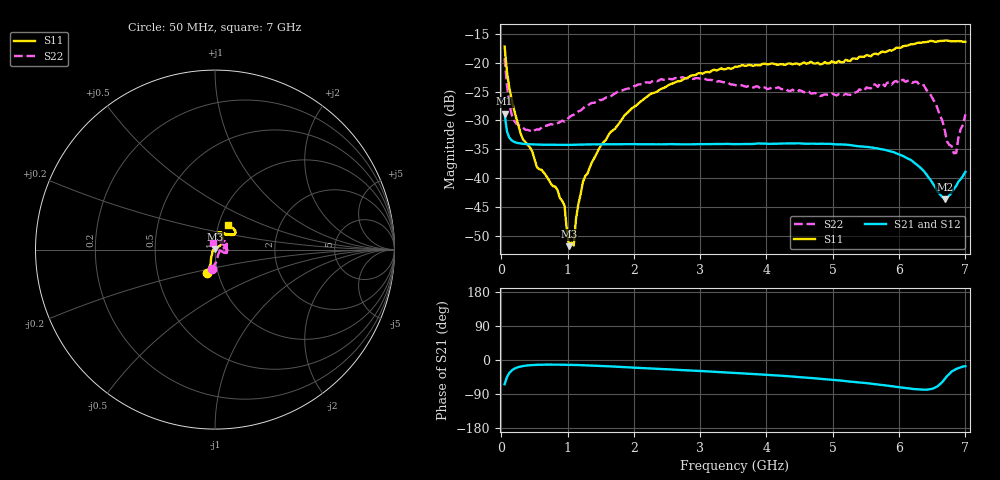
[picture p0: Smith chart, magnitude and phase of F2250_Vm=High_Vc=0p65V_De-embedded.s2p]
! Integrated Device Technology
! Corporate Headquarters
! 6024 Silver Creek Valley Road
! San Jose, CA 95138  USA
! Phone:  1-408-284-8200
! Toll Free:  1-800-223-1366
! Webpage:  http://www.idt.com/
! Timing and RF Division
! 515 Groton Road, Suite 102
! Westford, MA 01886-6024
! Device:  F2250
! Description: Voltage Variable RF Attenuator
! Frequency:  50.0 -  6000.00 MHz
! Package:  3x3 mm Thin QFN Plastic Package: 16 pin
! Ports:  2 RF, 3 DC
!  Pin  1  = GND
!  Pin  2  = NC
!  Pin  3  = RF1  = Port 1
!  Pin  4  = NC
!  Pin  5  = GND
!  Pin  6  = GND
!  Pin  7  = GND
!  Pin  8  = GND
!  Pin  9  = NC
!  Pin 10  = RF2  = Port 2
!  Pin 11  = NC
!  Pin 12  = GND
!  Pin 13  = GND
!  Pin 14  = VCNTRL
!  Pin 15  = VDD
!  Pin 16  = VMODE
! Vcntrl:  0.650 Volts
! Vmode:  +3.300 Volts
! Vdd:  +3.30  Volts
! Current:  1.282 mA
! Data:  The device was measured on a the F2250 evaluation board which has
!  individual transmission lines to the RF pins.  Data was collected
!  using a calibrated network analyzer.  The evaluation board was
!  de-embedded using a TRL calibration technique.
!  The reference plane is the edge of the package pin.
! Misc:  SN 10
!  Action Tracker AT0258
! Date Measured:  2014-11-26
! Date:  2015-10-15  MJV
! Note:
!  Integrated Device Technology supplies this data as a sample of measured
!  data at the package pin for this product.  Your particular data for this
!  product may vary.
!  Data was taken at 25 degrees C.
!  Integrated Device Technology reserves the right to change this data at anytime.
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# GHz S dB R 50
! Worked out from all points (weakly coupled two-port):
!   201 points, 50 MHz to 7 GHz, reference 50 ohm
!   highest |S21| = -28.81 dB at 50 MHz (marker M1); lowest = -43.7 dB at 6.687 GHz (marker M2)
!   lowest |S11| = -51.8 dB at 1.023 GHz (marker M3), VSWR 1.01, Z = 49.8 + j0.172 ohm
!   |S11| at or under -10 dB: start of sweep to end of sweep
!   |S22| runs from -35.7 to -19.2 dB; largest |S21 - S12| = 6.3e-05
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0.05  -17.17 -108.3  -28.81 -64.0  -28.81 -64.0  -19.20 -99.3
0.1195  -24.20 -111.6  -32.95 -34.6  -32.94 -34.6  -26.90 -70.8
0.22375  -29.45 -121.8  -33.84 -20.8  -33.83 -20.8  -30.51 -47.2
0.5365  -38.09 -153.6  -34.17 -12.7  -34.17 -12.7  -31.55 -9.8
0.8145  -41.46 170.6  -34.22 -12.2  -34.22 -12.2  -30.65 -1.3
0.9535  -44.77 171.5  -34.23 -12.5  -34.23 -12.5  -30.21 0.4
1.023  -51.81 137.7  -34.23 -12.7  -34.23 -12.7  -29.45 2.1
1.0925  -51.70 83.0  -34.22 -13.0  -34.21 -13.0  -29.01 3.5
1.12725  -47.04 56.6  -34.21 -13.2  -34.21 -13.2  -28.68 2.8
1.2315  -40.66 38.5  -34.17 -13.7  -34.17 -13.7  -27.89 2.2
1.6485  -31.98 40.4  -34.12 -16.9  -34.13 -16.9  -25.82 10.3
2.37825  -24.75 46.3  -34.13 -23.4  -34.13 -23.4  -23.05 20.7
3.525  -20.67 71.5  -34.10 -34.1  -34.10 -34.1  -23.83 48.6
4.7065  -20.09 71.9  -34.02 -48.0  -34.02 -48.0  -25.27 53.9
5.2625  -19.68 53.1  -34.26 -57.0  -34.26 -57.1  -25.56 29.1
5.85325  -17.81 40.4  -35.31 -68.4  -35.31 -68.4  -23.36 0.8
6.3745  -16.41 40.8  -38.79 -78.4  -38.79 -78.4  -23.89 -15.8
6.54825  -16.36 44.6  -41.66 -72.4  -41.67 -72.6  -27.01 -18.1
6.68725  -16.13 47.7  -43.69 -50.4  -43.69 -50.3  -31.58 0.5
6.722  -16.11 49.2  -43.43 -42.6  -43.41 -42.5  -33.62 6.1
6.861  -16.23 54.4  -41.35 -23.8  -41.33 -23.7  -35.63 64.3
7  -16.35 62.3  -38.92 -16.4  -38.89 -16.6  -28.93 106.5
